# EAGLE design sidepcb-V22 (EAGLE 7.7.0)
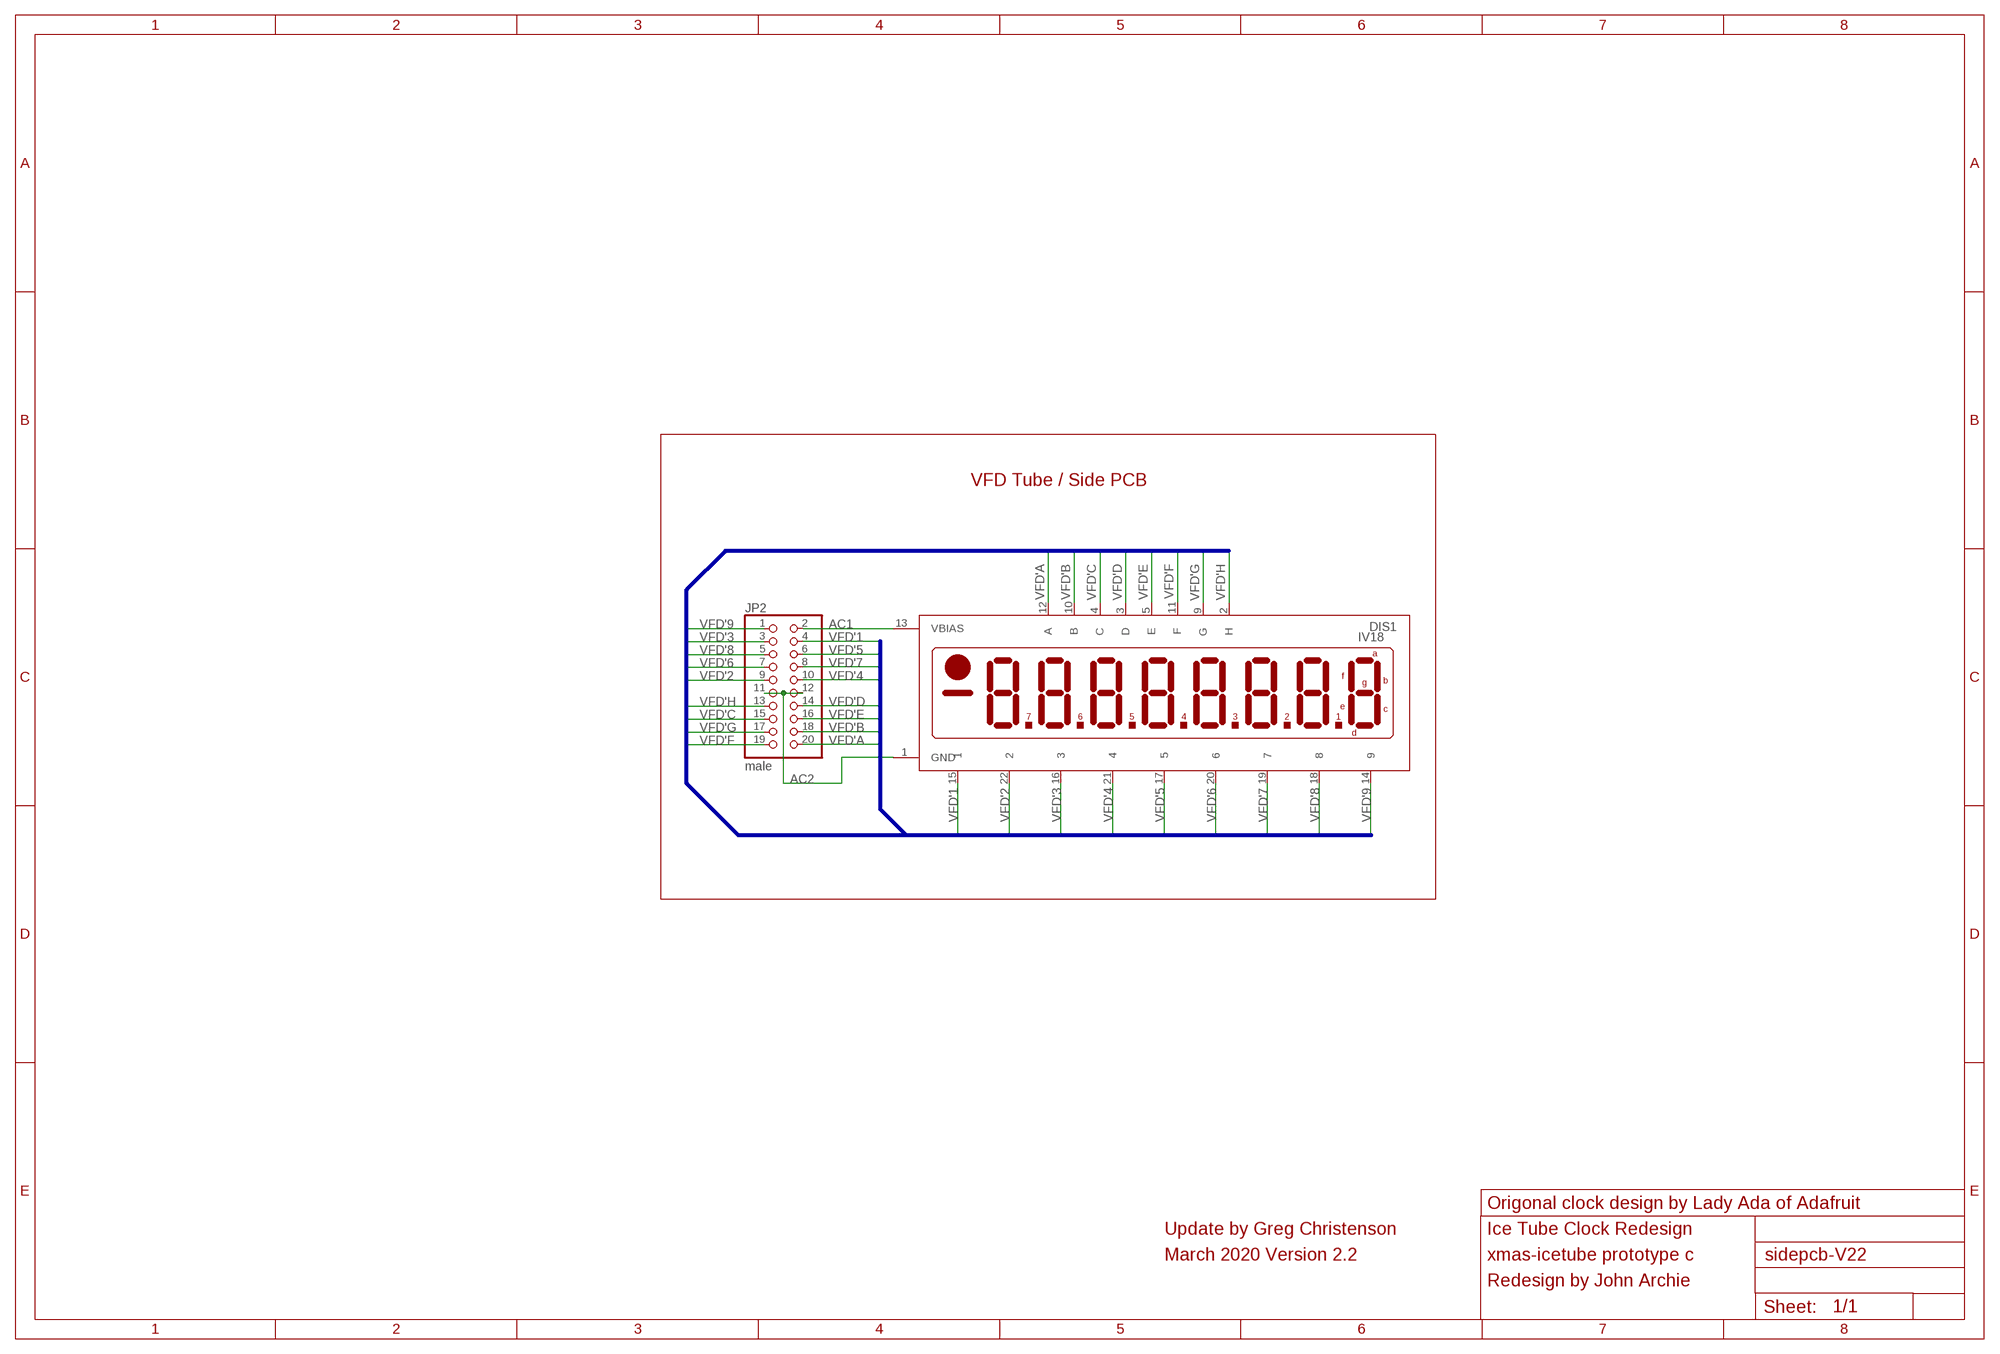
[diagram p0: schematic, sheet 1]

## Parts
DIS1  IV18  [IV18]
JP2  male  PINHD-2X10  [2X10]

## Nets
AC1: DIS1.13(VBIAS) JP2.2
AC2: DIS1.1(GND) JP2.11 JP2.12
VFD'1: DIS1.15 JP2.4
VFD'2: DIS1.22 JP2.9
VFD'3: DIS1.16 JP2.3
VFD'4: DIS1.21 JP2.10
VFD'5: DIS1.17 JP2.6
VFD'6: DIS1.20 JP2.7
VFD'7: DIS1.19 JP2.8
VFD'8: DIS1.18 JP2.5
VFD'9: DIS1.14 JP2.1
VFD'A: DIS1.12(A) JP2.20
VFD'B: DIS1.10(B) JP2.18
VFD'C: DIS1.4(C) JP2.15
VFD'D: DIS1.3(D) JP2.14
VFD'E: DIS1.5(E) JP2.16
VFD'F: DIS1.11(F) JP2.19
VFD'G: DIS1.9(G) JP2.17
VFD'H: DIS1.2(H) JP2.13

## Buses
VFD[1..9],VFD_A,VFD_B,VFD_C,VFD_D,VFD_E,VFD_F,VFD_G,VFD_H

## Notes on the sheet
- VFD Tube / Side PCB
- Origonal clock design by Lady Ada of Adafruit
- Update by Greg Christenson | Ice Tube Clock Redesign
- March 2020 Version 2.2 | xmas-icetube prototype c
- Redesign by John Archie

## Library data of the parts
DIS1 = vfd:IV18: LCD DISPLAY 8-character 7 segment
JP2 = pinhead:PINHD-2X10: PIN HEADER

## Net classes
0 default: clearance 0.205 mm

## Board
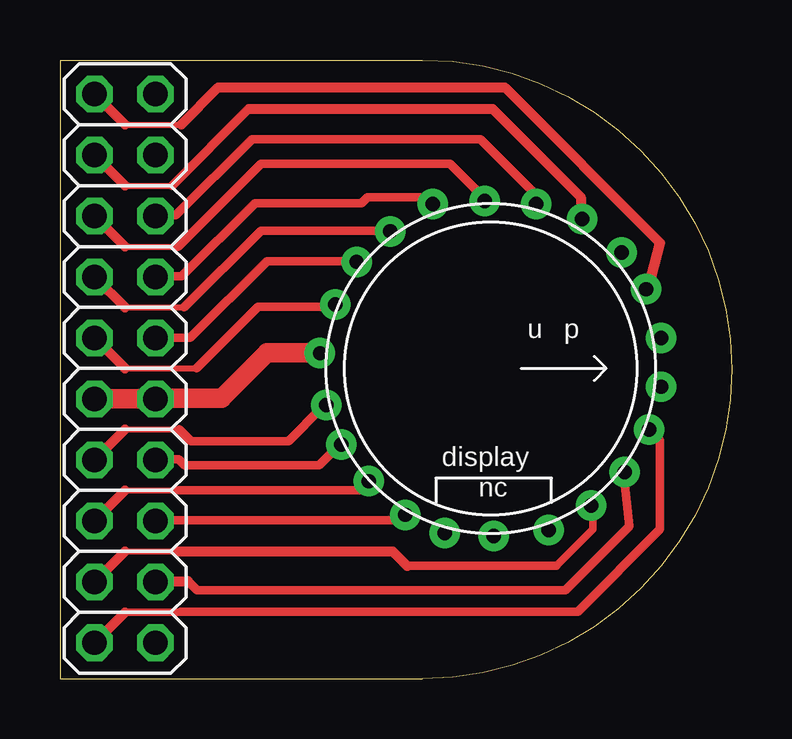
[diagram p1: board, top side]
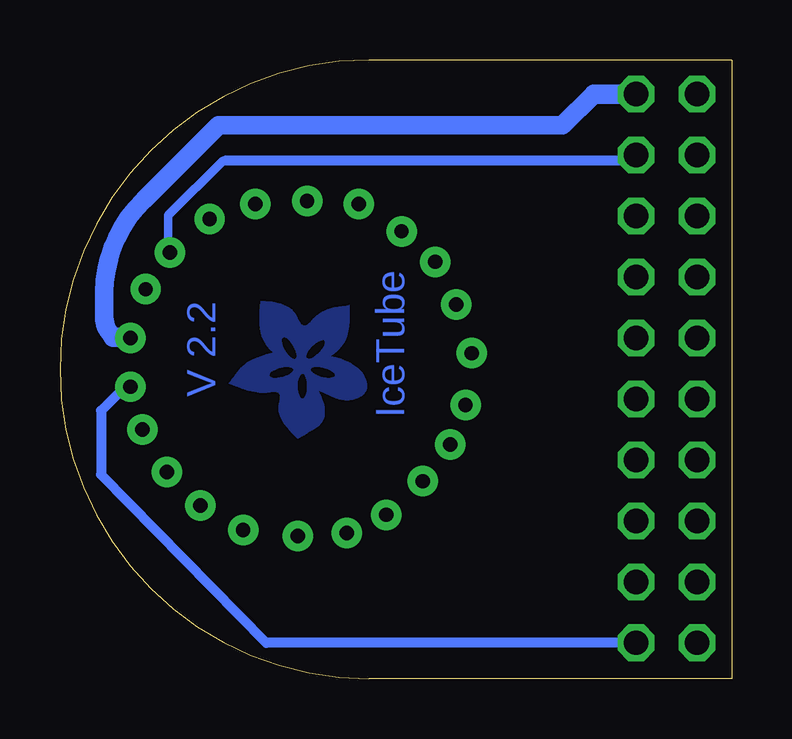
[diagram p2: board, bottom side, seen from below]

Size 28 x 25.78 mm. Coordinates in mm from the lower left corner, seen from the top.
Outline: 0,25.78 0,0 15.11,0 arc180 15.11,25.78 0,25.78
Copper layers (1*16): Top 0.0356mm / dielectric 1.5011mm / Bottom 0.0356mm
Design rules "LaenPCBOrder *": minimum track width 8mil, minimum drill 9mil, track to track 10mil, track to pad 10mil, pad to pad 10mil, via to via 10mil, smd to smd 8mil, copper to edge 15mil, drill to drill 6mil, minimum pad ring 7mil, minimum via ring 7mil, stop-mask expansion 4mil, vias tented up to drill 20mil, thermal gap 10mil

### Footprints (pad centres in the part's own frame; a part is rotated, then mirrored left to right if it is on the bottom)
IV18 = drill 0.6 pad 1.27: 1 -0.635,-7.112; 2 1.524,-6.858; 3 3.175,-6.223; 4 4.699,-5.08; 5 6.096,-3.556; 6 6.858,-1.905; 7 6.985,0.127; 8 6.731,2.413; 9 5.715,4.191; 10 4.318,5.588; 11 2.54,6.604; 12 0.762,7.112; 13 -1.27,7.112; 14 -3.302,6.477; 15 -4.826,5.461; 16 -6.223,3.81; 17 -6.858,1.905; 18 -6.985,-0.254; 19 -6.858,-2.413; 20 -5.715,-4.191; 21 -4.445,-5.588; 22 -2.667,-6.477
2X10 = drill 1.016 octagon: 1 -11.43,-1.27; 2 -11.43,1.27; 3 -8.89,-1.27; 4 -8.89,1.27; 5 -6.35,-1.27; 6 -6.35,1.27; 7 -3.81,-1.27; 8 -3.81,1.27; 9 -1.27,-1.27; 10 -1.27,1.27; 11 1.27,-1.27; 12 1.27,1.27; 13 3.81,-1.27; 14 3.81,1.27; 15 6.35,-1.27; 16 6.35,1.27; 17 8.89,-1.27; 18 8.89,1.27; 19 11.43,-1.27; 20 11.43,1.27

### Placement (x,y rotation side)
DIS1  17.95,12.93 270 top
JP2  2.71,12.93 270 top

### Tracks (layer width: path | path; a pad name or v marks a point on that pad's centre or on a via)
AC1
  Bottom 0.254: 25.09,14.22 DIS1.13 25.07,14.27
  Bottom 0.61: 25.8,14.25 25.78,14.22 | 25.13,14.22 arc45 DIS1.13
  Bottom 0.762: 5.74,24.36 7.06,23.06 21.39,23.06 24.51,19.94 arc-45 26.16,16.11 26.16,15.11 arc-45 25.8,14.25
  Bottom 0.813: JP2.2 5.74,24.36 | 25.78,14.22 25.13,14.22
AC2
  Top 0.254: DIS1.1 10.92,13.52 10.67,13.46 10.54,13.59 | 4.01,11.68 JP2.12
  Top 0.813: 10.54,13.59 8.64,13.59 6.73,11.68 4.01,11.68 | JP2.11 JP2.12
N$6
  cutout Bottom: 17,14.08 16.97,14.05 16.96,14.01 16.97,13.96 17,13.88 17.05,13.78 17.16,13.64 17.24,13.56 17.34,13.48 17.45,13.4 17.54,13.36 17.62,13.34 17.67,13.35 17.7,13.37 17.71,13.39 17.72,13.42 17.72,13.47 17.71,13.51 17.67,13.58 17.62,13.69 17.52,13.8 17.45,13.87 17.34,13.96 17.27,14.02 17.19,14.06 17.11,14.09 17.06,14.1 17.02,14.1
N$7
  cutout Bottom: 18.17,13.37 18.16,13.4 18.15,13.46 18.16,13.53 18.18,13.63 18.24,13.77 18.29,13.86 18.36,13.98 18.43,14.06 18.49,14.13 18.56,14.18 18.61,14.2 18.65,14.22 18.69,14.21 18.72,14.18 18.74,14.14 18.75,14.11 18.75,14.07 18.74,14.02 18.73,13.98 18.69,13.86 18.66,13.79 18.61,13.68 18.56,13.6 18.51,13.53 18.42,13.43 18.37,13.39 18.31,13.35 18.26,13.33 18.23,13.32 18.2,13.34 18.18,13.35
N$8
  cutout Bottom: 18.29,12.87 18.29,12.9 18.3,12.92 18.33,12.94 18.37,12.96 18.43,12.98 18.49,12.98 18.53,12.98 18.61,12.98 18.68,12.97 18.77,12.95 18.86,12.93 18.96,12.9 19.04,12.86 19.11,12.83 19.18,12.78 19.22,12.74 19.25,12.69 19.26,12.65 19.25,12.61 19.22,12.58 19.17,12.56 19.12,12.55 19.08,12.54 18.95,12.54 18.85,12.56 18.76,12.57 18.69,12.59 18.62,12.62 18.54,12.65 18.46,12.69 18.4,12.73 18.37,12.75 18.33,12.78 18.31,12.81 18.3,12.84 18.29,12.86
N$11
  cutout Bottom: 18.08,12.19 18.07,12.06 18.06,11.94 18.02,11.83 17.99,11.76 17.96,11.71 17.91,11.68 17.88,11.69 17.85,11.7 17.81,11.74 17.78,11.8 17.75,11.86 17.74,11.91 17.73,11.97 17.72,12.04 17.71,12.1 17.71,12.3 17.72,12.38 17.73,12.44 17.74,12.48 17.76,12.53 17.78,12.58 17.8,12.61 17.81,12.64 17.84,12.66 17.86,12.68 17.88,12.69 17.91,12.69 17.94,12.68 17.97,12.64 17.99,12.61 18.02,12.57 18.03,12.52 18.05,12.45 18.07,12.36
N$13
  cutout Bottom: 16.79,12.54 16.72,12.55 16.66,12.56 16.62,12.57 16.59,12.59 16.57,12.61 16.56,12.63 16.56,12.66 16.57,12.69 16.58,12.72 16.61,12.76 16.66,12.8 16.75,12.85 16.85,12.89 16.91,12.92 16.99,12.94 17.05,12.96 17.15,12.97 17.22,12.98 17.27,12.98 17.32,12.98 17.38,12.98 17.43,12.97 17.48,12.95 17.51,12.93 17.52,12.92 17.53,12.89 17.53,12.86 17.51,12.82 17.48,12.78 17.44,12.75 17.4,12.72 17.35,12.69 17.3,12.66 17.26,12.64 17.2,12.62 17.11,12.59 17.01,12.57 16.94,12.55 16.87,12.54
N$14
  pour Bottom: 230 corners
VFD'1
  Bottom 0.254: JP2.4 3.96,21.59 | 23.49,17.84 DIS1.15
  Bottom 0.356: 21.08,21.59 21.21,21.59 23.49,19.3 23.49,17.84
  Bottom 0.406: 3.96,21.59 20.83,21.59 21.08,21.59
VFD'2
  Top 0.254: 2.71,12.93 5.69,12.93 | 11.56,15.49 11.56,15.52 DIS1.22
  Top 0.356: 5.69,12.93 8.26,15.49 11.56,15.49
  Top 0.406: JP2.9 2.71,12.93
VFD'3
  Top 0.254: 2.71,20.55 4.67,20.55 | 21.72,19.3 21.76,19.26 DIS1.16
  Top 0.356: 4.67,20.55 7.87,23.75
  Top 0.406: JP2.3 2.71,20.55 | 7.87,23.75 18.03,23.75 21.72,20.07 21.72,19.3
VFD'4
  Top 0.254: 12.57,17.53 12.39,17.4 DIS1.21
  Top 0.356: JP2.10 5.44,14.2 8.64,17.4 12.39,17.4
VFD'5
  Top 0.254: DIS1.17 19.88,19.81 19.94,19.81 19.94,20.07 | 4.19,19.3 4.17,19.28 JP2.6
  Top 0.356: 19.94,20.07 17.53,22.48 8,22.48 4.83,19.3 4.19,19.3
VFD'6
  Top 0.254: 2.71,15.47 5.18,15.47 | 13.97,18.67 13.84,18.56 DIS1.20
  Top 0.356: 5.18,15.47 8.38,18.67 13.97,18.67
  Top 0.406: JP2.7 2.71,15.47
VFD'7
  Top 0.254: 15.52,19.81 DIS1.19 | 4.19,16.76 4.17,16.74 JP2.8
  Top 0.356: 15.52,19.81 15.26,20.07 12.83,20.07 12.57,19.81 8.13,19.81 5.08,16.76 4.19,16.76
VFD'8
  Top 0.254: 2.71,18.01 4.93,18.01 | 17.65,19.87 17.65,19.81 | 17.65,19.87 DIS1.18 | 17.65,20.07 17.65,19.87
  Top 0.356: 4.93,18.01 8.38,21.46 16.26,21.46 17.65,20.07
  Top 0.406: JP2.5 2.71,18.01
VFD'9
  Top 0.254: 2.71,23.09 5.06,23.09 | 24.51,16.26 24.46,16.26 DIS1.14
  Top 0.406: JP2.1 2.71,23.09 | 5.06,23.09 6.6,24.64 18.54,24.64 25.02,18.16 24.51,16.26
VFD'A
  Bottom 0.254: 25.27,12.19 25.25,12.17 DIS1.12
  Bottom 0.406: JP2.20 19.41,1.5 26.29,8.51 26.29,11.18 25.27,12.19
VFD'B
  Top 0.254: JP2.18 4.01,4.06 | 23.49,8.64 23.52,8.64 DIS1.10
  Top 0.356: 5.33,4.06 5.72,3.68 21.08,3.68 23.75,6.35 23.49,8.64
  Top 0.406: 4.01,4.06 5.33,4.06
VFD'C
  Top 0.254: 12.83,8.15 DIS1.4 | 2.71,7.85 4.95,7.85
  Top 0.356: 12.83,8.15 12.55,7.85 4.95,7.85
  Top 0.406: JP2.15 2.71,7.85
VFD'D
  Top 0.254: JP2.14 4.01,9.14 | DIS1.3 11.63,9.65 11.56,9.65
  Top 0.356: 4.01,9.14 4.95,9.14 5.21,8.89 10.8,8.89 11.56,9.65
VFD'E
  Top 0.254: JP2.16 4.01,6.6
  Top 0.305: 14.17,6.6 DIS1.5
  Top 0.356: 4.01,6.6 14.17,6.6
VFD'F
  Top 0.305: 2.71,2.77 5,2.77 5.03,2.79
  Top 0.356: DIS1.11 25.02,9.93 25.02,6.22 21.59,2.79 5.03,2.79
  Top 0.406: JP2.19 2.71,2.77
VFD'G
  Top 0.254: 2.71,5.31 4.9,5.31 | 22.23,7.13 DIS1.9
  Top 0.305: 20.7,4.7 22.23,6.22 22.23,7.13
  Top 0.356: 14.48,4.7 20.7,4.7
  Top 0.406: JP2.17 2.71,5.31 | 4.9,5.31 13.87,5.31 14.48,4.7
VFD'H
  Top 0.254: 2.71,10.39 4.98,10.39 | 10.92,11.3 11.07,11.43 DIS1.2
  Top 0.356: 4.98,10.39 5.46,9.91 9.53,9.91 10.92,11.3
  Top 0.406: JP2.13 2.71,10.39

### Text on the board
Bottom: IceTube | V 2.2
